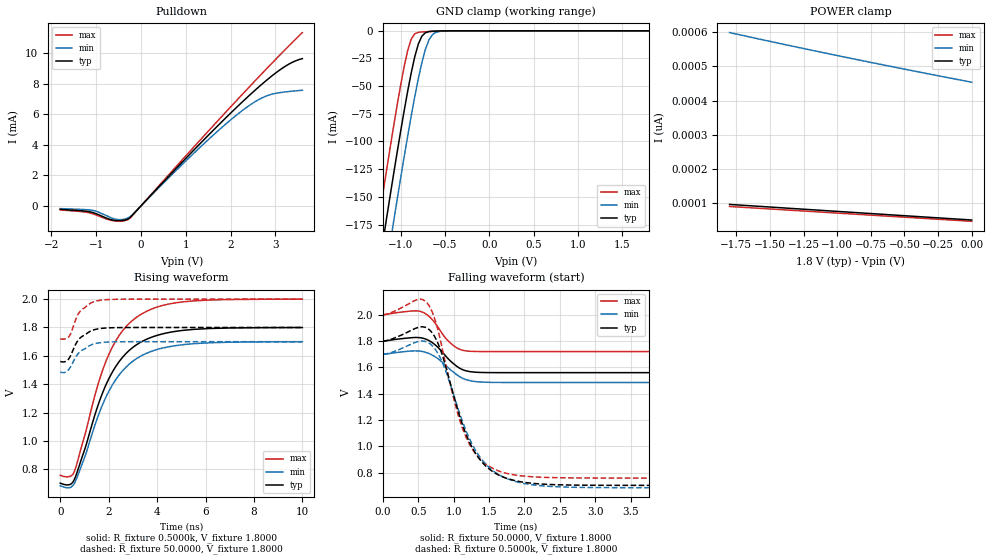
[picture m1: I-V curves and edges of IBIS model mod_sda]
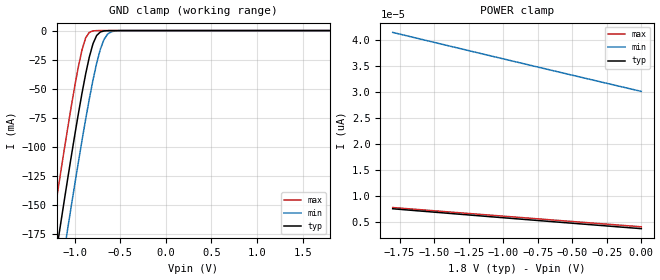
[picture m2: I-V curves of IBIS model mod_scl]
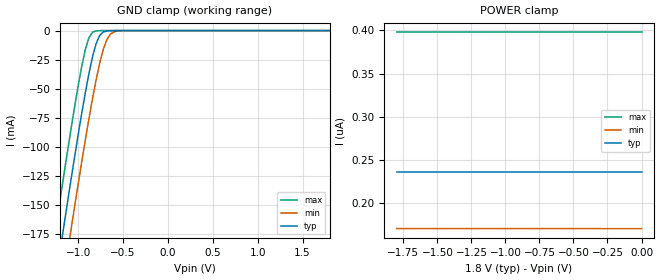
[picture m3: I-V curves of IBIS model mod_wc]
| IBIS (I/O, Buffer, Information, Specification) Model, officially
| electronic behavioral standard for Buffer structures of digital pins.
[IBIS ver]  4.0
[File name] m24c16_fc1_tssop8.ibs
[File Rev]  1.0
[Date]   10 April 2014
[Source]   CAD & Design Services (Catania) - STMicroelectronics
[Notes]
   (Note1)  This IBIS model includes the TSSOP8 package data
   (Note2)  This IBIS model has some Notes about the non-monotonicity
   of the I-V curves, but they are not indicative of problems
   inside the model;
[Copyright] (c) 2014 STMicroelectronics
|   Component M24C16
[Component] M24C16
[Manufacturer] STMicroelectronics
[Package]
| variable   typ   min   max
R_pkg   0.0   0.0   0.0
L_pkg   0.0H   0.0H   0.0H
C_pkg   0.0F   0.0F   0.0F
[Pin]  signal_name   model_name   R_pin   L_pin   C_pin
1   1NC   NC   NA   NA   NA
2   2NC   NC   NA   NA   NA
3   3NC   NC   NA   NA   NA
4   VSS   GND   NA   NA   NA
5   SDA   mod_sda   NA   NA   NA
6   SCL   mod_scl   NA   NA   NA
7   WCN   mod_wc   NA   NA   NA
8   VCC   POWER   NA   NA   NA
[Package Model]  182696_TSSOP8
[Define Package Model]  182696_TSSOP8
[Manufacturer]  STMicroelectronics
[OEM]  STMicroelectronics
[Description]  8 pin TSSOP package
[Number Of Pins]  8
[Pin Numbers]
|Pin Num   Terminal Name
1   | net1
2   | net2
3   | net3
4   | net4_GND
5   | net5
6   | net6
7   | net7
8   | net8_VDD
[Model Data]
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[End Model Data]
[End Package Model]
| Models and submodels in the file (3): mod_sda (I/O_open_drain), mod_scl (Input), mod_wc (Input)
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|   Model mod_sda
[Model]   mod_sda
Model_type I/O_open_drain
Polarity   Non-Inverting
Vinl   =   0.540V
Vinh   =   1.260V
Vmeas  =   0.900V
Cref   =   10pF
Rref   =   1k
Vref   =   1.800V
C_comp   1.845pF   1.683pF   1.932pF
[Temperature Range]  25.0000   85.0000   -40.0000
[Voltage Range]   1.8000V   1.7000V   2.0000V
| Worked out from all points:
|   slope of the pulldown table from 0 to 0.27 V, typ, clamps not added: 318 ohm
|   GND clamp passes 1 mA (typ) near -0.69 V on its own axis
|   rising waveform, R_fixture 0.5000k, V_fixture 1.8000: 20-80 % time 1.56ns typ, 1.57ns min, 1.51ns max; typ from 0.702 V to 1.8 V
|   rising waveform, R_fixture 50.0000, V_fixture 1.8000: 20-80 % time 609ps typ, 634ps min, 568ps max; typ from 1.56 V to 1.8 V
|   falling waveform, R_fixture 50.0000, V_fixture 1.8000: 20-80 % time 267ps typ, 290ps min, 246ps max; typ from 1.8 V to 1.56 V
|   falling waveform, R_fixture 0.5000k, V_fixture 1.8000: 20-80 % time 438ps typ, 480ps min, 398ps max; typ from 1.8 V to 0.703 V
[Pulldown]
|Voltage   I(typ)   I(min)   I(max)
-1.8V     -222uA     -177.7uA   -265uA
-1.08V    -428uA     -290uA     -513uA
-540mV    -965uA     -880.2uA   -1.003mA
-360mV    -928uA     -862uA     -966uA
-240mV    -759.3uA   -706.6uA   -792.3uA
1.32V     4.078mA    3.84mA     4.308mA
1.92V     5.844mA    5.429mA    6.226mA
2.34V     7.023mA    6.413mA    7.548mA
2.64V     7.819mA    6.98mA     8.479mA
2.88V     8.413mA    7.278mA    9.214mA
3.3V      9.281mA    7.487mA    10.47mA
3.6V      9.641mA    7.571mA    11.35mA
[GND_clamp]
|Voltage   I(typ)   I(min)   I(max)
-1.8V     -510.8mA   -553.4mA   -468.4mA
-1.28V    -232.9mA   -276.2mA   -189.3mA
-1.24V    -212mA     -255.4mA   -168.4mA
-1.16V    -170.7mA   -214mA     -127.2mA
-1.08V    -130.3mA   -173.4mA   -87.22mA
-920mV    -54.71mA   -95.34mA   -17.95mA
-840mV    -23.48mA   -59.58mA   -2.706mA
-800mV    -12mA      -43.3mA    -1.362mA
-720mV    -1.701mA   -16.74mA   -836.3uA
-680mV    -666.5uA   -8.196mA   -697.4uA
-600mV    -197.9uA   -1.292mA   -438.8uA
1.8V      51.71pA    461.1pA    43.15pA
[POWER_clamp]
|Voltage   I(typ)   I(min)   I(max)
-1.8V     97.17pA    598.3pA    91.12pA
-1.42V    87.5pA     565.9pA    81.99pA
-980mV    76.35pA    529.7pA    71.43pA
-480mV    63.75pA    490.1pA    59.44pA
0V        51.71pA    453.6pA    47.94pA
[Ramp]
| variable   typ   min   max
dV/dt_r  0.1438/0.6835n   0.1288/0.7046n   0.1678/0.6305n
dV/dt_f  0.1438/0.3076n   0.1288/0.3432n   0.1678/0.2726n
R_load = 50.0000
[Rising Waveform]
R_fixture= 0.5000k
V_fixture= 1.8000
V_fixture_min= 1.7000
V_fixture_max= 2.0000
|time   V(typ)   V(min)   V(max)
0s        702.4mV    684.3mV    757.6mV
560ps     720.9mV    694.7mV    776.8mV
1.02ns    945.2mV    890.6mV    1.044V
1.52ns    1.231V     1.155V     1.375V
1.9ns     1.4V       1.314V     1.567V
2.44ns    1.561V     1.467V     1.746V
3.14ns    1.677V     1.579V     1.871V
3.98ns    1.743V     1.644V     1.943V
5.07ns    1.78V      1.679V     1.981V
10ns      1.8V       1.7V       2V
[Rising Waveform]
R_fixture= 50.0000
V_fixture= 1.8000
V_fixture_min= 1.7000
V_fixture_max= 2.0000
|time   V(typ)   V(min)   V(max)
0s        1.56V      1.485V     1.72V
210ps     1.56V      1.484V     1.72V
370ps     1.584V     1.508V     1.738V
450ps     1.61V      1.531V     1.765V
690ps     1.698V     1.605V     1.877V
850ps     1.73V      1.634V     1.919V
1.25ns    1.774V     1.675V     1.971V
1.59ns    1.791V     1.691V     1.99V
2.63ns    1.8V       1.7V       2V
10ns      1.8V       1.7V       2V
[Falling Waveform]
R_fixture= 50.0000
V_fixture= 1.8000
V_fixture_min= 1.7000
V_fixture_max= 2.0000
|time   V(typ)   V(min)   V(max)
0s        1.8V       1.7V       2V
420ps     1.827V     1.725V     2.029V
570ps     1.821V     1.72V      2.018V
730ps     1.776V     1.684V     1.943V
870ps     1.698V     1.625V     1.834V
970ps     1.641V     1.576V     1.778V
1.09ns    1.593V     1.528V     1.737V
1.25ns    1.567V     1.497V     1.722V
1.73ns    1.56V      1.486V     1.72V
10ns      1.56V      1.485V     1.72V
[Falling Waveform]
R_fixture= 0.5000k
V_fixture= 1.8000
V_fixture_min= 1.7000
V_fixture_max= 2.0000
|time   V(typ)   V(min)   V(max)
0s        1.8V       1.7V       2V
480ps     1.901V     1.794V     2.114V
640ps     1.894V     1.789V     2.08V
820ps     1.726V     1.663V     1.792V
1.02ns    1.351V     1.359V     1.324V
1.18ns    1.086V     1.112V     1.065V
1.42ns    868.8mV    885.3mV    880.8mV
1.76ns    754.7mV    753mV      793.1mV
2.84ns    704.7mV    687.7mV    759.7mV
10ns      702.6mV    684.5mV    758.1mV
|   Model mod_scl
[Model]   mod_scl
Model_type Input
Vinl   =   0.540V
Vinh   =   1.260V
C_comp   1.762pF   1.683pF   1.932pF
[Temperature Range]  25.0000   85.0000   -40.0000
[Voltage Range]   1.8000V   1.7000V   2.0000V
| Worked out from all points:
|   GND clamp passes 1 mA (typ) near -0.71 V on its own axis
[GND_clamp]
|Voltage   I(typ)   I(min)   I(max)
-1.8V     -506.7mA   -549.3mA   -463.8mA
-1.28V    -230.6mA   -274mA     -186.5mA
-1.24V    -209.8mA   -253.3mA   -165.8mA
-1.16V    -168.9mA   -212.2mA   -124.8mA
-1.08V    -128.7mA   -171.8mA   -85.14mA
-920mV    -53.64mA   -94.29mA   -16.44mA
-840mV    -22.68mA   -58.76mA   -1.468mA
-800mV    -11.31mA   -42.6mA    -261.9uA
-720mV    -1.249mA   -16.25mA   -6.98uA
-680mV    -318.6uA   -7.797mA   -1.128uA
-600mV    -18.77uA   -1.043mA   -29.45nA
1.8V      3.674pA    30.76pA    3.627pA
[POWER_clamp]
|Voltage   I(typ)   I(min)   I(max)
-1.8V     7.509pA    41.51pA    7.748pA
-940mV    5.652pA    36.04pA    5.962pA
-440mV    4.594pA    32.89pA    4.934pA
0V        3.674pA    30.14pA    4.034pA
|   Model mod_wc
[Model]   mod_wc
Model_type Input
Vinl   =   0.540V
Vinh   =   1.260V
C_comp   1.762pF   1.683pF   1.932pF
[Temperature Range]  25.0000   85.0000   -40.0000
[Voltage Range]   1.8000V   1.7000V   2.0000V
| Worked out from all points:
|   GND clamp passes 1 mA (typ) near -0.71 V on its own axis
[GND_clamp]
|Voltage   I(typ)   I(min)   I(max)
-1.8V     -506.7mA   -549.3mA   -463.8mA
-1.28V    -230.6mA   -274mA     -186.5mA
-1.24V    -209.8mA   -253.3mA   -165.8mA
-1.16V    -168.9mA   -212.2mA   -124.8mA
-1.08V    -128.7mA   -171.8mA   -85.14mA
-920mV    -53.64mA   -94.29mA   -16.44mA
-840mV    -22.68mA   -58.76mA   -1.468mA
-800mV    -11.31mA   -42.6mA    -261.9uA
-720mV    -1.249mA   -16.25mA   -6.98uA
-680mV    -318.6uA   -7.797mA   -1.128uA
-600mV    -18.77uA   -1.043mA   -29.45nA
1.8V      3.674pA    30.76pA    3.627pA
[POWER_clamp]
|Voltage   I(typ)   I(min)   I(max)
-1.8V     235.8nA    170.8nA    397.7nA
-300mV    235.8nA    170.8nA    397.7nA
-280mV    235.8nA    170.7nA    397.7nA
0V        235.8nA    170.7nA    397.7nA
